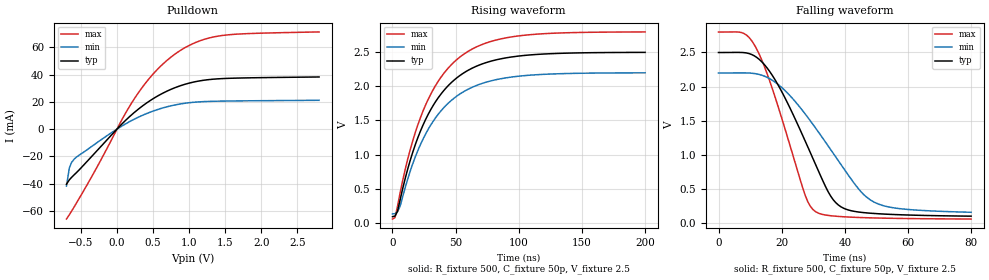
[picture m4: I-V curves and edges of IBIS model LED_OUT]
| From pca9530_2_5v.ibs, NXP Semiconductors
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[Model]   LED_OUT
Model_type Open_drain
Vref=2.5
Vmeas=1.25
Rref=500
Cref=50p
C_comp   5p   4.8p   5.2p
[Temperature Range] 27   85   -40
[Voltage Range]   2.5   2.2   2.8
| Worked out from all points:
|   slope of the pulldown table from 0 to 0.375 V, typ, clamps not added: 21 ohm
|   falling waveform, R_fixture 500, C_fixture 50p, V_fixture 2.5: 20-80 % time 14.5ns typ, 19.1ns min, 11.2ns max; typ from 2.5 V to 0.102 V
|   rising waveform, R_fixture 500, C_fixture 50p, V_fixture 2.5: 20-80 % time 35.4ns typ, 35.5ns min, 35.4ns max; typ from 0.088 V to 2.5 V
[Pulldown]
-700mV    -40.51mA   -41.9mA    -66.09mA
-660mV    -37.29mA   -28.54mA   -62.93mA
-630mV    -35.54mA   -24.61mA   -60.4mA
-560mV    -31.91mA   -20.52mA   -54.22mA
-280mV    -16.06mA   -10.08mA   -28.24mA
80mV      4.386mA    2.619mA    8.045mA
250mV     12.66mA    7.552mA    23.06mA
500mV     22.32mA    13.24mA    40.43mA
780mV     29.92mA    17.48mA    54.2mA
1.07V     34.66mA    19.74mA    63.22mA
1.42V     37mA       20.54mA    68.49mA
2.8V      38.3mA     21.15mA    71.41mA
[Falling Waveform]
R_fixture=500
C_fixture=50p
V_fixture=2.5
V_fixture_min=2.2
V_fixture_max=2.8
0s        2.5V       2.2V       2.8V
8.081ns   2.498V     2.201V     2.778V
12.12ns   2.428V     2.186V     2.548V
18.59ns   2.047V     2.043V     1.75V
27.47ns   1.2V       1.598V     405mV
30.71ns   862.4mV    1.395V     168.4mV
34.75ns   457.4mV    1.129V     112.4mV
37.98ns   264.5mV    912.2mV    98.01mV
49.29ns   141mV      307.5mV    75.58mV
80ns      101.7mV    158.7mV    59.68mV
[Rising Waveform]
R_fixture=500
C_fixture=50p
V_fixture=2.5
V_fixture_min=2.2
V_fixture_max=2.8
0s        88.31mV    129.4mV    53.93mV
2.02ns    97.05mV    132.3mV    76.39mV
6.061ns   336.5mV    242.1mV    439.8mV
14.14ns   920.8mV    762.1mV    1.079V
24.24ns   1.435V     1.229V     1.641V
38.38ns   1.887V     1.641V     2.134V
54.55ns   2.175V     1.902V     2.447V
72.73ns   2.34V      2.054V     2.627V
98.99ns   2.443V     2.148V     2.738V
200ns     2.499V     2.199V     2.799V
[Ramp]
R_load=500
dV/dt_r   1.447E+0/1.533E-9   1.411E+0/2.501E-9   1.471E+0/1.002E-9
dV/dt_f   1.440E+0/1.196E-8   1.393E+0/1.761E-8   1.469E+0/8.565E-9
|[End   LED_OUT
